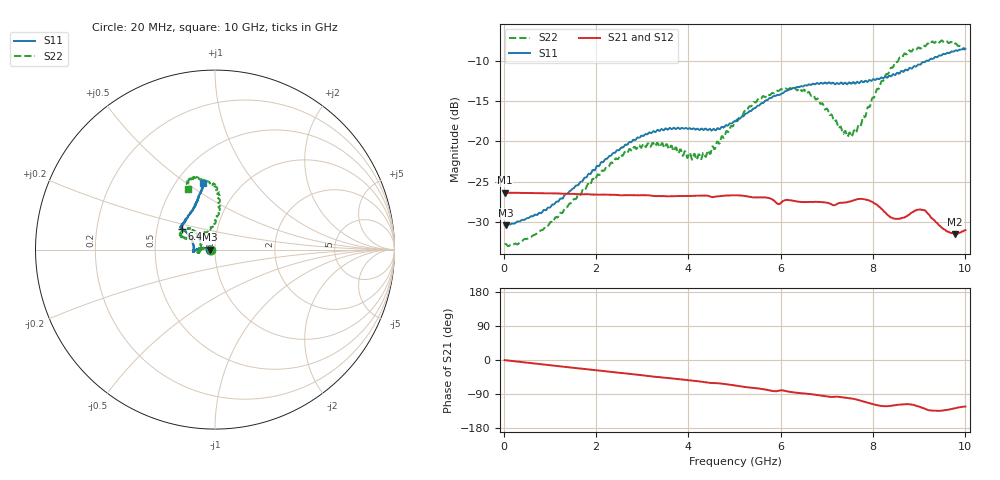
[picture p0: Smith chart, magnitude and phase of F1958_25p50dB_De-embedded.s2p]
! Integrated Device Technology
! Corporate Headquarters
! 6024 Silver Creek Valley Road
! San Jose, CA 95138  USA
! Phone:  1-408-284-8200
! Toll Free:  1-800-223-1366
! Webpage:  http://www.idt.com/
! Timing and RF Division
! 515 Groton Road, Suite 102
! Westford, MA 01886-6024
! Device:  F1958
! Description: 7-bit 0.25 dB Digital Step Attenuator
! Frequency:  0.001 -  6.000 GHz
! Package:  4x4 mm Thin QFN Plastic Package: 24 pin
! Ports:  2 RF, 12 DC
!  Pin  1  = D0
!  Pin  2  = VDD
!  Pin  3  = VMODE
!  Pin  4  = GND
!  Pin  5  = RF1  =  Port 1
!  Pin  6  = GND
!  Pin  7  = GND
!  Pin  8  = GND
!  Pin  9  = GND
!  Pin 10  = GND
!  Pin 11  = GND
!  Pin 12  = GND
!  Pin 13  = GND
!  Pin 14  = RF2  =  Port 2
!  Pin 15  = GND
!  Pin 16  = LE
!  Pin 17  = CLK
!  Pin 18  = DATA
!  Pin 19  = D6
!  Pin 20  = D5
!  Pin 21  = D4
!  Pin 22  = D3
!  Pin 23  = D2
!  Pin 24  = D1
! State:  102
! Atten State:  25.50 dB
! Voltage:  +3.30 Volts
! Current:  0.258 mA
! Data:  The device was measured on a F1958 evaluation board which has
!  individual transmission lines to the RF pins.  Data was collected
!  using a calibrated network analyzer.  The evaluation board was
!  de-embedded using Automatic Fixture Removal (AFR).
!  The reference plane is the edge of the package pin.
! Misc:
!  Action Tracker AT0419
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# GHz S dB R 50
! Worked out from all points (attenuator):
!   500 points, 20 MHz to 10 GHz, reference 50 ohm
!   highest |S21| = -26.35 dB at 20 MHz (marker M1); lowest = -31.5 dB at 9.78 GHz (marker M2)
!   lowest |S11| = -30.4 dB at 40 MHz (marker M3), VSWR 1.06, Z = 47.1 - j0.043 ohm
!   |S11| at or under -10 dB: start of sweep to 9.154 GHz
!   |S22| runs from -33.0 to -7.5 dB; largest |S21 - S12| = 0.00031
!   S11 on the Smith chart (normalised r, x): 20 MHz: 0.94, -0.00; 6.4 GHz: 0.67, +0.16; 10 GHz: 0.67, +0.58
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0.02  -30.37 -178.9  -26.35 -0.3  -26.35 -0.3  -32.74 -178.7
0.04  -30.40 -179.1  -26.36 -0.5  -26.35 -0.5  -32.70 -178.2
0.32  -29.91 175.2  -26.37 -4.5  -26.37 -4.5  -32.67 174.7
0.84  -28.72 171.0  -26.42 -11.5  -26.41 -11.5  -30.98 172.9
1.7  -24.96 171.1  -26.55 -22.9  -26.54 -22.9  -26.12 172.2
2.6  -20.66 177.0  -26.66 -34.8  -26.63 -34.8  -21.53 -179.7
3.36  -18.67 -175.4  -26.77 -45.2  -26.76 -45.3  -20.51 -168.5
4.24  -18.58 -178.7  -26.73 -56.5  -26.73 -56.5  -21.63 169.8
4.5  -18.65 175.4  -26.88 -60.6  -26.89 -60.6  -21.02 152.2
5.02  -17.52 161.0  -26.67 -67.5  -26.68 -67.4  -17.43 138.7
5.58  -15.26 150.7  -26.94 -76.2  -26.94 -76.2  -14.68 140.3
5.94  -14.22 148.5  -27.75 -81.7  -27.76 -81.8  -13.73 149.1
6.4  -13.26 148.0  -27.48 -87.2  -27.50 -87.1  -13.41 156.1
6.68  -12.89 146.9  -27.49 -90.5  -27.51 -90.4  -14.32 158.1
7.5  -12.72 138.6  -27.45 -101.0  -27.45 -100.9  -18.89 120.7
7.68  -12.68 135.7  -27.14 -105.5  -27.14 -105.4  -17.97 100.6
7.9  -12.49 129.3  -27.28 -113.3  -27.28 -113.3  -15.69 90.1
8.34  -11.87 119.4  -29.22 -121.7  -29.21 -121.8  -11.48 84.3
8.66  -11.38 113.6  -29.45 -116.9  -29.48 -117.1  -9.27 87.9
9.1  -10.18 107.6  -28.51 -127.6  -28.51 -127.7  -8.12 100.4
9.78  -8.71 100.6  -31.45 -127.5  -31.44 -127.5  -7.86 111.8
10  -8.50 100.2  -31.00 -122.9  -31.02 -122.9  -8.63 113.8
